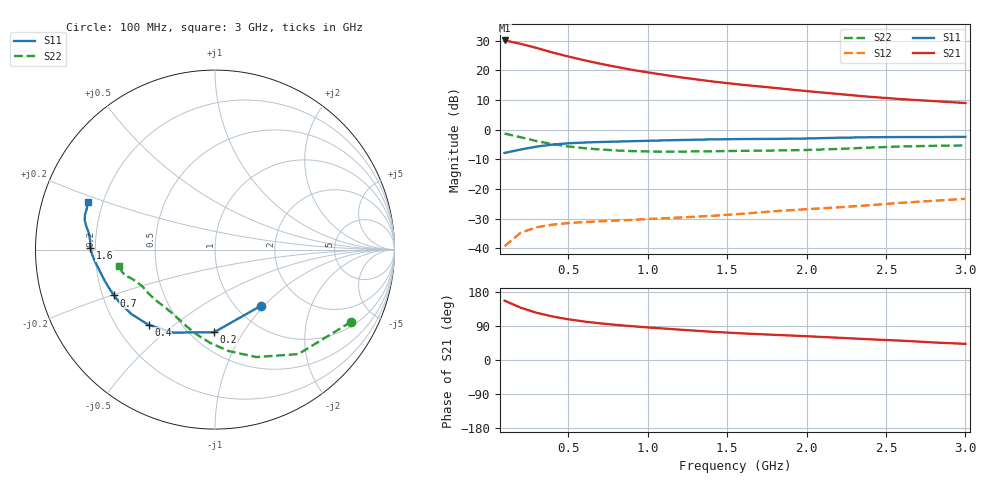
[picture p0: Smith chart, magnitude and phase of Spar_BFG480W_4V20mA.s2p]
! Filename: 420BFG480.001
! Title: BFG480W
! Bias: Vce=4V; Ic=20mA
! Company: NXP Semiconductors NL
! User: Quality&Reliability T&D
! Measure time: 10 Nov 1999 / 12:02:24
#  MHz  S  MA  R 50
! Freq  S11  S21  S12  S22  :
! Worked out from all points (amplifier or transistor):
!   20 points, 100 MHz to 3 GHz, reference 50 ohm
!   highest |S21| = 30.1 dB at 100 MHz (marker M1)
!   |S21| within 3 dB of that: start of sweep to 332.3 MHz
!   unconditionally stable (mu >= 1): 1.358 GHz to end of sweep
!   at 400 MHz: K = 0.40, MSG = 29.1 dB, |S12| = -32.1 dB
!   at 1.2 GHz: K = 0.94, MSG = 23.7 dB, |S12| = -29.7 dB
!   at 3 GHz: K = 1.10, MAG = 14.3 dB, |S12| = -23.3 dB
!   S11 on the Smith chart (normalised r, x): 100 MHz: 1.29, -0.96; 200 MHz: 0.64, -0.75; 400 MHz: 0.33, -0.41; 700 MHz: 0.25, -0.20; 1.6 GHz: 0.18, +0.01; 3 GHz: 0.14, +0.18
100  0.4046 -50.5  31.99 156.5  0.0108 63.8  0.8583 -28.0
200  0.4609 -90.7  28.11 138.3  0.01812 53.6  0.7449 -51.4
300  0.517 -116.6  23.98 124.7  0.02243 46.5  0.642 -68.9
400  0.5595 -131.4  20.08 115.0  0.02492 42.2  0.5705 -82.3
500  0.5879 -142.3  17.18 107.5  0.02646 40.1  0.521 -92.9
600  0.6057 -149.9  14.84 101.6  0.02754 39.4  0.487 -101.2
700  0.6185 -155.6  12.99 96.8  0.02838 39.9  0.463 -108.0
800  0.6285 -160.3  11.5 92.7  0.02921 40.8  0.4459 -113.8
900  0.6379 -164.1  10.24 89.2  0.02995 42.5  0.4344 -118.9
1000  0.6479 -167.7  9.252 86.1  0.03097 44.2  0.4277 -123.6
1200  0.6676 -173.3  7.685 80.2  0.03286 47.8  0.4256 -131.7
1400  0.6843 -177.4  6.539 74.6  0.03501 51.5  0.4321 -138.0
1600  0.6942 179.2  5.698 70.2  0.03812 55.5  0.4385 -142.9
1800  0.6978 175.7  5.06 66.4  0.04199 59.1  0.4447 -147.6
2000  0.7087 172.6  4.474 62.8  0.04541 62.3  0.4533 -152.9
2200  0.7297 169.6  3.995 58.8  0.04881 64.4  0.4721 -157.9
2400  0.7445 167.2  3.58 54.6  0.05299 65.9  0.4981 -161.6
2600  0.7501 165.1  3.267 50.9  0.0584 67.1  0.5206 -164.0
2800  0.7498 162.5  3.033 46.3  0.06292 67.1  0.5326 -166.5
3000  0.7557 159.6  2.813 42.6  0.06805 67.5  0.5415 -170.0
